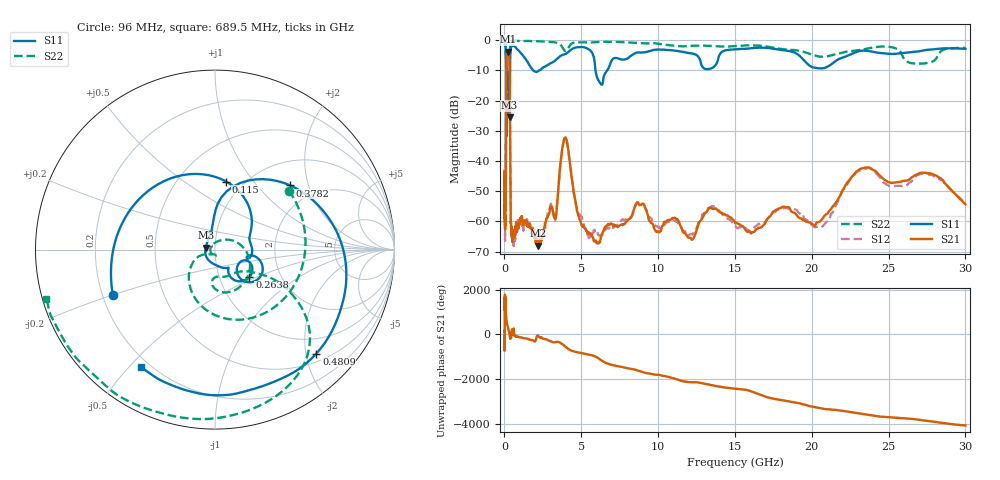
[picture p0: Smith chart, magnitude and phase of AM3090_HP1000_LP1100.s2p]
! Date/Time: Thu, Feb 28, 2019 2:02 PM
! Network Analyzer: Agilent Technologies E8364B Rev: A.07.50.67
! Sweep from 0.010 to 30.000 GHz, 1601 Points, Sweep Type: LOG
! Power Supply: 5.023 V, 0.002 A
# Hz S DB R 50
!freq MagS11 AngS11 MagS21 AngS21 MagS12 AngS12 MagS22 AngS22
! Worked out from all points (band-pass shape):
!   1601 points, 10 MHz to 30 GHz, reference 50 ohm
!   highest |S21| = -3.81 dB at 225.9 MHz (marker M1); lowest = -68.1 dB at 2.18 GHz (marker M2)
!   |S21| within 3 dB of the highest: 123.3 MHz to 323.7 MHz (200.3 MHz wide, 89.6 % of centre)
!   lowest |S11| = -25.6 dB at 333.7 MHz (marker M3), VSWR 1.11, Z = 45.1 + j1.02 ohm
!   |S11| at or under -10 dB: 118.2 MHz to 360.9 MHz (242.7 MHz wide, 101 % of centre); 1.865 GHz to 2.255 GHz (390.8 MHz wide, 19 % of centre); 5.925 GHz to 6.695 GHz (769.8 MHz wide, 12.2 % of centre)
!   |S22| runs from -31.7 to -0.1 dB; largest |S21 - S12| = 0.013
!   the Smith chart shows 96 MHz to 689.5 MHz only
!   S11 on the Smith chart (normalised r, x): 96 MHz: 0.24, -0.20; 115 MHz: 0.83, +0.74; 263.8 MHz: 1.39, -0.46; 378.2 MHz: 1.50, +1.54; 480.9 MHz: 0.66, -2.21; 689.5 MHz: 0.17, -0.54
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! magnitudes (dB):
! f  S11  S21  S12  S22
! 10 MHz  -0.2  -43.7  -43.1  -0.6
! 38.04 MHz  -0.5  -58.7  -60.0  -1.5
! 84.29 MHz  -2.5  -54.0  -52.8  -4.6
! 96 MHz  -4.1  -38.8  -39.2  -5.6
! 115 MHz  -8.3  -12.2  -12.2  -9.5
! 144.7 MHz  -14.1  -4.3  -4.3  -31.7
! 225.9 MHz  -16.2  -3.8  -3.8  -15.2
! 263.8 MHz  -12.2  -4.1  -4.1  -16.1
! 333.7 MHz  -25.6  -8.6  -8.6  -9.7
! 378.2 MHz  -5.2  -40.8  -41.3  -1.1
! 480.9 MHz  -1.8  -64.6  -65.2  -0.2
! 550.5 MHz  -1.9  -64.0  -63.8  -0.2
! 689.5 MHz  -2.2  -63.6  -65.5  -0.2
! 2.084 GHz  -10.6  -66.5  -65.7  -0.4
! 2.18 GHz  -10.3  -68.1  -63.3  -0.4
! 3.302 GHz  -6.8  -59.1  -59.8  -0.8
! 3.934 GHz  -4.7  -32.3  -32.2  -3.6
! 5.392 GHz  -2.8  -63.9  -64.3  -0.8
! 7.926 GHz  -6.3  -60.1  -59.5  -0.8
! 20.31 GHz  -9.2  -60.5  -61.8  -5.2
! 23.48 GHz  -3.5  -42.2  -42.6  -3.0
! 30 GHz  -2.9  -54.4  -53.7  -2.6
